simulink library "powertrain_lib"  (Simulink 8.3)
settings: Solver=ode45  StartTime=0.0  StopTime=10.0  RelTol=1e-3
libraries: electric_lib x4, controls_lib x4, vehicle_lib x4, engine_lib x4, transmission_lib x4, accessory_lib x1, powertrain_lib x1

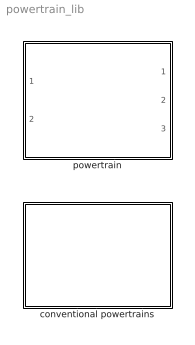
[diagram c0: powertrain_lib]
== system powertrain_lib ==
  conventional powertrains : Subsystem
  powertrain : Subsystem  Variant=on

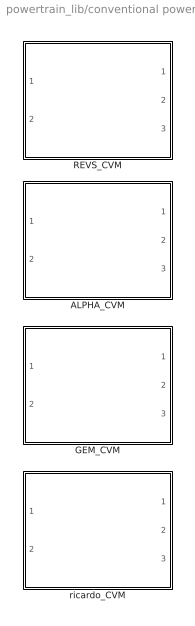
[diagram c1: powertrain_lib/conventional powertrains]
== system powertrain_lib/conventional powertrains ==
  ALPHA_CVM : Subsystem  VariantControl=vehicle_powertrain_type == enum_powertrain_type.conventional && REVS_current_model_type == enum_model_type.ALPHA
  GEM_CVM : Subsystem
  REVS_CVM : Subsystem
  ricardo_CVM : Subsystem

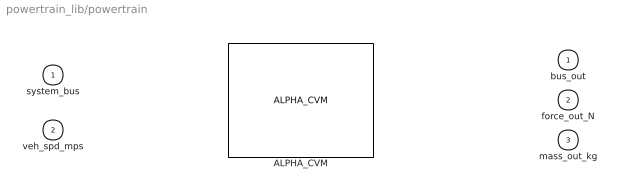
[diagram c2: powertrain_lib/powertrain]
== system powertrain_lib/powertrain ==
  system_bus : Inport
  veh_spd_mps : Inport  Port=2
  ALPHA_CVM : powertrain_lib/conventional powertrains/ALPHA_CVM  VariantControl=vehicle_powertrain_type == enum_powertrain_type.conventional && REVS_current_model_type == enum_model_type.ALPHA
  bus_out : Outport
  force_out_N : Outport  Port=2
  mass_out_kg : Outport  Port=3

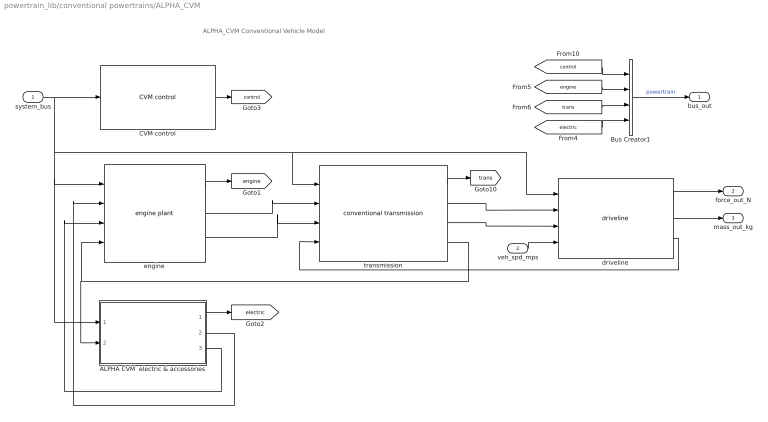
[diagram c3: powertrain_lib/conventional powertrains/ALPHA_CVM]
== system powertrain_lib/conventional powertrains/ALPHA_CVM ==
  note: ALPHA_CVM Conventional Vehicle Model
  system_bus : Inport
  veh_spd_mps : Inport  Port=2
  ALPHA CVM  electric & accessories : Subsystem  VariantControl=variants_electric_ALPHA
  Bus Creator1 : BusCreator
  CVM control : controls_lib/CVM control
  driveline : vehicle_lib/driveline variants/driveline
  engine : engine_lib/engine plant  SystemSampleTime=-1
  transmission : transmission_lib/conventional transmission
  bus_out : Outport
  force_out_N : Outport  Port=2
  mass_out_kg : Outport  Port=3
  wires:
  CVM control/1 -> [control]
  ALPHA CVM  electric & accessories/2(trq_out_Nm) -> engine/2
  transmission/4 -> ALPHA CVM  electric & accessories/2(spd_in_radps), engine/4
  engine/3 -> transmission/3
  ALPHA CVM  electric & accessories/3(iner_out_kgm2) -> engine/3
  driveline/3 -> transmission/4
  transmission/3 -> driveline/3
  ALPHA CVM  electric & accessories/1(bus_out) -> [electric]
  transmission/2 -> driveline/2
  engine/1 -> [engine]
  transmission/1 -> [trans]
  engine/2 -> transmission/2
  Bus Creator1/1 -> bus_out/1  "powertrain"
  [electric] -> Bus Creator1/4
  [control] -> Bus Creator1/1
  [engine] -> Bus Creator1/2
  [trans] -> Bus Creator1/3
  system_bus/1 -> CVM control/1, engine/1, ALPHA CVM  electric & accessories/1(system_bus), transmission/1, driveline/1
  veh_spd_mps/1 -> driveline/4
  driveline/1 -> force_out_N/1
  driveline/2 -> mass_out_kg/1

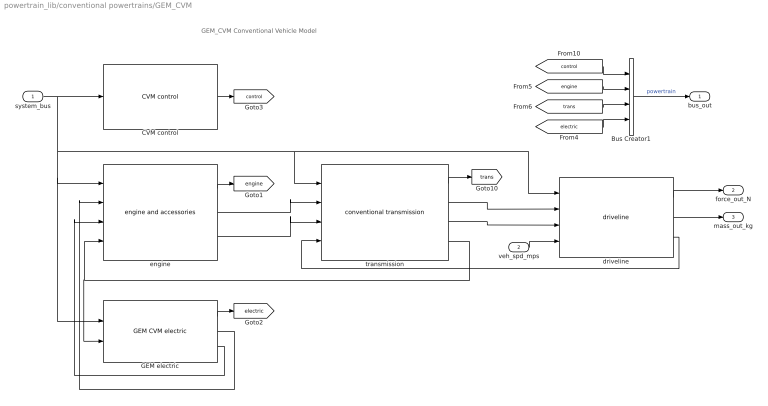
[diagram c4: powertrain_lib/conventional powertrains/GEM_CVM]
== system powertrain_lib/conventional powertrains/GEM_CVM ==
  note: GEM_CVM Conventional Vehicle Model
  system_bus : Inport
  veh_spd_mps : Inport  Port=2
  Bus Creator1 : BusCreator
  CVM control : controls_lib/CVM control
  GEM electric : electric_lib/GEM CVM electric  VariantControl=variants_electric_GEM
  driveline : vehicle_lib/driveline variants/driveline
  engine : engine_lib/engine and accessories
  transmission : transmission_lib/conventional transmission
  bus_out : Outport
  force_out_N : Outport  Port=2
  mass_out_kg : Outport  Port=3
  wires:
  CVM control/1 -> [control]
  GEM electric/2 -> engine/2
  transmission/4 -> GEM electric/2, engine/4
  engine/3 -> transmission/3
  GEM electric/3 -> engine/3
  driveline/3 -> transmission/4
  transmission/3 -> driveline/3
  GEM electric/1 -> [electric]
  transmission/2 -> driveline/2
  engine/1 -> [engine]
  transmission/1 -> [trans]
  engine/2 -> transmission/2
  Bus Creator1/1 -> bus_out/1  "powertrain"
  [electric] -> Bus Creator1/4
  [control] -> Bus Creator1/1
  [engine] -> Bus Creator1/2
  [trans] -> Bus Creator1/3
  system_bus/1 -> CVM control/1, GEM electric/1, engine/1, transmission/1, driveline/1
  veh_spd_mps/1 -> driveline/4
  driveline/1 -> force_out_N/1
  driveline/2 -> mass_out_kg/1

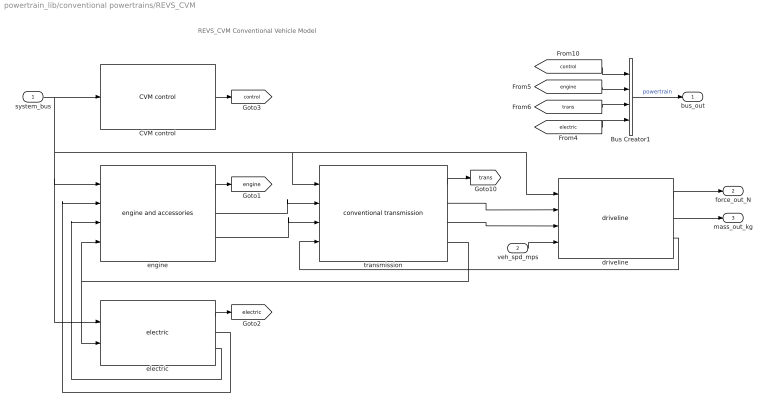
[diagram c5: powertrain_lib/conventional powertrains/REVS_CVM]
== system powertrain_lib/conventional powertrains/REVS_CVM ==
  note: REVS_CVM Conventional Vehicle Model
  system_bus : Inport
  veh_spd_mps : Inport  Port=2
  Bus Creator1 : BusCreator
  CVM control : controls_lib/CVM control
  driveline : vehicle_lib/driveline variants/driveline
  electric : electric_lib/electric
  engine : engine_lib/engine and accessories
  transmission : transmission_lib/conventional transmission
  bus_out : Outport
  force_out_N : Outport  Port=2
  mass_out_kg : Outport  Port=3
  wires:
  driveline/2 -> mass_out_kg/1
  driveline/1 -> force_out_N/1
  veh_spd_mps/1 -> driveline/4
  system_bus/1 -> driveline/1, transmission/1, electric/1, engine/1, CVM control/1
  [trans] -> Bus Creator1/3
  [engine] -> Bus Creator1/2
  [control] -> Bus Creator1/1
  [electric] -> Bus Creator1/4
  Bus Creator1/1 -> bus_out/1  "powertrain"
  engine/2 -> transmission/2
  transmission/1 -> [trans]
  engine/1 -> [engine]
  transmission/2 -> driveline/2
  electric/1 -> [electric]
  transmission/3 -> driveline/3
  driveline/3 -> transmission/4
  electric/3 -> engine/3
  engine/3 -> transmission/3
  transmission/4 -> electric/2, engine/4
  electric/2 -> engine/2
  CVM control/1 -> [control]

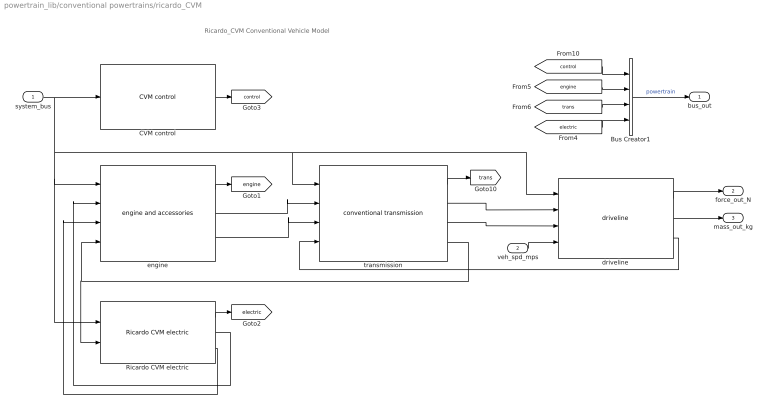
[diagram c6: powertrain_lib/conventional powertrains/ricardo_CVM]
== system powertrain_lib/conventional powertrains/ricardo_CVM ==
  note: Ricardo_CVM Conventional Vehicle Model
  system_bus : Inport
  veh_spd_mps : Inport  Port=2
  Bus Creator1 : BusCreator
  CVM control : controls_lib/CVM control
  Ricardo CVM electric : electric_lib/Ricardo CVM electric  VariantControl=variants_electric_ALPHA_RICARDO
  driveline : vehicle_lib/driveline variants/driveline
  engine : engine_lib/engine and accessories
  transmission : transmission_lib/conventional transmission
  bus_out : Outport
  force_out_N : Outport  Port=2
  mass_out_kg : Outport  Port=3
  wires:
  CVM control/1 -> [control]
  Ricardo CVM electric/2 -> engine/2
  transmission/4 -> Ricardo CVM electric/2, engine/4
  engine/3 -> transmission/3
  Ricardo CVM electric/3 -> engine/3
  driveline/3 -> transmission/4
  transmission/3 -> driveline/3
  Ricardo CVM electric/1 -> [electric]
  transmission/2 -> driveline/2
  engine/1 -> [engine]
  transmission/1 -> [trans]
  engine/2 -> transmission/2
  Bus Creator1/1 -> bus_out/1  "powertrain"
  [electric] -> Bus Creator1/4
  [control] -> Bus Creator1/1
  [engine] -> Bus Creator1/2
  [trans] -> Bus Creator1/3
  system_bus/1 -> CVM control/1, Ricardo CVM electric/1, engine/1, transmission/1, driveline/1
  veh_spd_mps/1 -> driveline/4
  driveline/1 -> force_out_N/1
  driveline/2 -> mass_out_kg/1

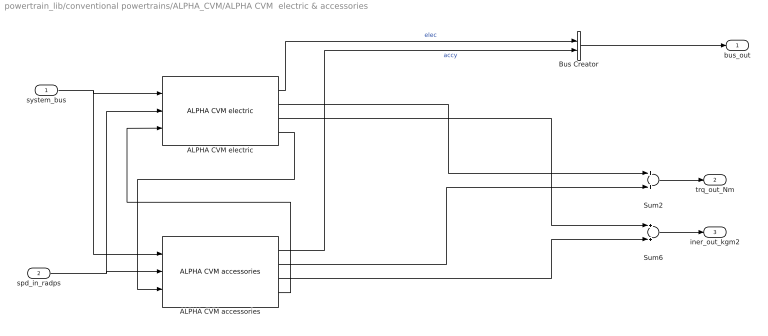
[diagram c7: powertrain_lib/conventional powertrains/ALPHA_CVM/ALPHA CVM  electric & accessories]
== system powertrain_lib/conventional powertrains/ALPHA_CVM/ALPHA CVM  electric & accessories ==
  system_bus : Inport
  spd_in_radps : Inport  Port=2
  ALPHA CVM accessories : accessory_lib/ALPHA CVM accessories  VariantControl=variants_electric_ALPHA
  ALPHA CVM electric : electric_lib/ALPHA CVM electric  VariantControl=variants_electric_ALPHA
  Bus Creator : BusCreator  Inputs=2
  Sum2 : Sum
  Sum6 : Sum
  bus_out : Outport
  trq_out_Nm : Outport  Port=2
  iner_out_kgm2 : Outport  Port=3
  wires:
  ALPHA CVM electric/2 -> Sum2/1
  ALPHA CVM accessories/2 -> Sum2/2
  ALPHA CVM accessories/3 -> Sum6/2
  ALPHA CVM electric/4 -> ALPHA CVM accessories/3
  ALPHA CVM accessories/1 -> Bus Creator/2  "accy"
  ALPHA CVM electric/1 -> Bus Creator/1  "elec"
  ALPHA CVM electric/3 -> Sum6/1
  ALPHA CVM accessories/4 -> ALPHA CVM electric/3
  Sum2/1 -> trq_out_Nm/1
  Sum6/1 -> iner_out_kgm2/1
  system_bus/1 -> ALPHA CVM accessories/1, ALPHA CVM electric/1
  Bus Creator/1 -> bus_out/1
  spd_in_radps/1 -> ALPHA CVM electric/2, ALPHA CVM accessories/2
